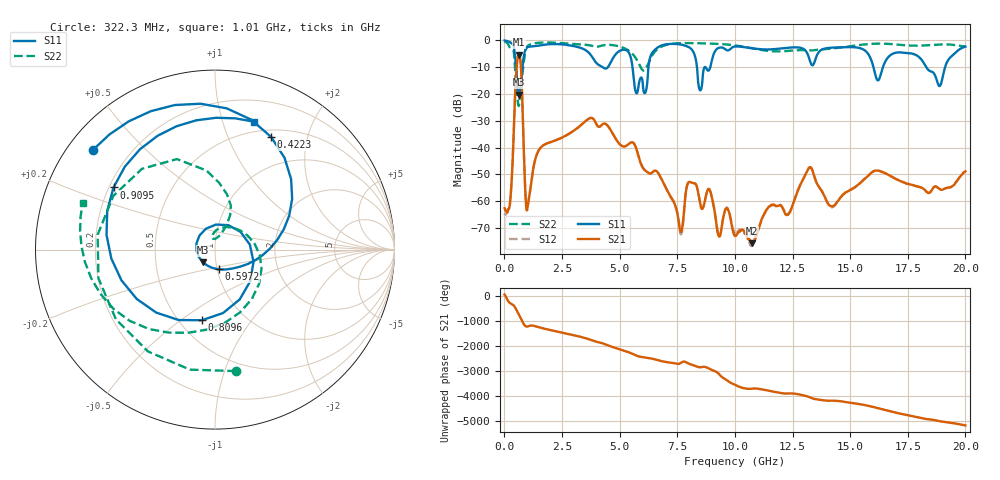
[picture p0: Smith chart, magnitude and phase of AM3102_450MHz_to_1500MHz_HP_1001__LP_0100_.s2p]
!Agilent Technologies,E8364B,MY43040894,A.07.50.67
!Agilent E8364B: A.07.50.67
!Date: Thursday, January 11, 2018 06:01:59
!Correction: S11(Full 2 Port(1,2))
!S21(Full 2 Port(1,2))
!S12(Full 2 Port(1,2))
!S22(Full 2 Port(1,2))
!S2P File: Measurements: S11, S21, S12, S22:
# Hz S  dB  R 50
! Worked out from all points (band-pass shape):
!   1601 points, 10 MHz to 20 GHz, reference 50 ohm
!   highest |S21| = -5.36 dB at 622.2 MHz (marker M1); lowest = -75.7 dB at 10.74 GHz (marker M2)
!   |S21| within 3 dB of the highest: 549.4 MHz to 704.3 MHz (155 MHz wide, 24.7 % of centre)
!   lowest |S11| = -20.2 dB at 634.7 MHz (marker M3), VSWR 1.22, Z = 43.3 - j6.1 ohm
!   |S11| at or under -10 dB: 5.558 GHz to 6.25 GHz (691.6 MHz wide, 11.7 % of centre); 16.01 GHz to 16.42 GHz (411.2 MHz wide, 2.54 % of centre); 18.3 GHz to 19.12 GHz (816.6 MHz wide, 4.36 % of centre)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
!   |S22| runs from -24.5 to -0.4 dB; largest |S21 - S12| = 0.0014
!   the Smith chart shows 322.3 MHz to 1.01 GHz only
!   S11 on the Smith chart (normalised r, x): 322.3 MHz: 0.07, +0.35; 422.3 MHz: 0.59, +1.45; 597.2 MHz: 1.01, -0.23; 809.6 MHz: 0.64, -0.60; 909.5 MHz: 0.22, +0.27; 1.01 GHz: 0.40, +1.27
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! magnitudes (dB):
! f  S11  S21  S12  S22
! 10 MHz  -0.1  -62.6  -65.2  -0.4
! 322.3 MHz  -1.1  -51.4  -51.1  -3.3
! 422.3 MHz  -3.1  -29.9  -29.8  -5.2
! 597.2 MHz  -19.0  -5.6  -5.6  -23.8
! 622.2 MHz  -20.1  -5.4  -5.4  -24.5
! 634.7 MHz  -20.2  -5.4  -5.4  -24.3
! 809.6 MHz  -8.0  -31.8  -32.0  -10.1
! 909.5 MHz  -3.6  -56.6  -56.8  -4.2
! 1.01 GHz  -2.6  -61.9  -61.9  -2.1
! 1.534 GHz  -1.9  -40.4  -40.4  -0.9
! 3.346 GHz  -2.9  -31.4  -31.4  -1.5
! 5.732 GHz  -19.8  -40.6  -40.6  -7.1
! 6.682 GHz  -2.5  -49.6  -49.6  -3.1
! 7.656 GHz  -1.6  -71.4  -72.4  -1.1
! 7.994 GHz  -2.5  -52.9  -52.9  -1.0
! 8.493 GHz  -18.7  -60.8  -60.9  -1.1
! 10.01 GHz  -2.3  -72.9  -72.1  -1.9
! 10.74 GHz  -3.0  -75.7  -76.3  -3.0
! 13.34 GHz  -9.2  -48.0  -48.0  -3.8
! 14.2 GHz  -2.7  -62.0  -62.3  -3.1
! 16.68 GHz  -6.1  -50.2  -50.2  -1.3
! 20 GHz  -2.4  -48.9  -48.9  -2.3
